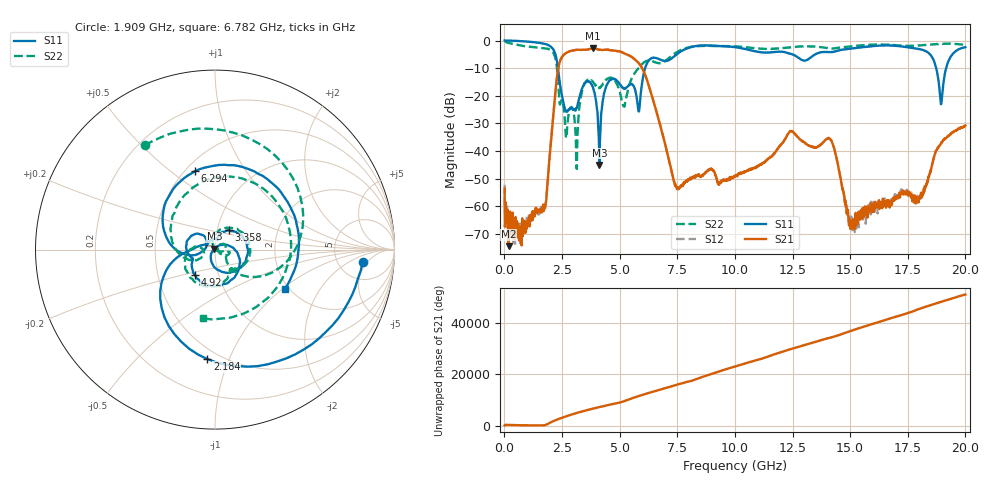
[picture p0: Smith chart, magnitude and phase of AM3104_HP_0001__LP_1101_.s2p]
!Created with skrf (http://scikit-rf.org).
# Hz S RI R 50.0
!freq ReS11 ImS11 ReS21 ImS21 ReS12 ImS12 ReS22 ImS22
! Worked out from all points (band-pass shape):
!   1601 points, 10 MHz to 20 GHz, reference 50 ohm
!   highest |S21| = -2.89 dB at 3.833 GHz (marker M1); lowest = -74.5 dB at 184.9 MHz (marker M2)
!   |S21| within 3 dB of the highest: 2.507 GHz to 5.513 GHz (3.006 GHz wide, 75 % of centre)
!   lowest |S11| = -45.0 dB at 4.12 GHz (marker M3), VSWR 1.01, Z = 49.7 + j0.448 ohm
!   |S11| at or under -10 dB: 2.323 GHz to 6.106 GHz (3.783 GHz wide, 89.8 % of centre); 18.74 GHz to 19.17 GHz (429.1 MHz wide, 2.26 % of centre)
!   |S22| runs from -46.5 to -0.2 dB; largest |S21 - S12| = 0.0069
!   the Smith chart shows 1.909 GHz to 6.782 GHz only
!   S11 on the Smith chart (normalised r, x): 1.909 GHz: 8.88, -3.80; 2.184 GHz: 0.43, -0.83; 3.358 GHz: 1.14, +0.25; 4.92 GHz: 0.77, -0.22; 6.294 GHz: 0.56, +0.61; 6.782 GHz: 1.90, -1.04
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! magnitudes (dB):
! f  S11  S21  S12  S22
! 10 MHz  0.0  -53.6  -52.2  -0.2
! 184.9 MHz  0.0  -74.5  -64.1  -0.9
! 1.909 GHz  -1.7  -47.5  -47.5  -3.1
! 2.184 GHz  -4.3  -21.1  -21.1  -5.6
! 2.684 GHz  -25.8  -4.5  -4.5  -35.3
! 3.346 GHz  -17.9  -3.4  -3.4  -19.2
! 3.358 GHz  -17.5  -3.4  -3.4  -18.6
! 3.833 GHz  -16.7  -2.9  -2.9  -14.9
! 4.12 GHz  -45.0  -3.4  -3.3  -17.1
! 4.92 GHz  -14.9  -3.9  -3.9  -16.6
! 5.82 GHz  -25.5  -8.1  -8.1  -10.0
! 6.294 GHz  -6.9  -17.1  -17.1  -7.3
! 6.682 GHz  -6.7  -28.3  -28.3  -8.2
! 6.782 GHz  -7.0  -31.4  -31.4  -8.2
! 7.506 GHz  -4.8  -53.3  -53.6  -4.0
! 10.01 GHz  -2.4  -49.2  -49.2  -2.1
! 13.34 GHz  -5.8  -38.6  -38.4  -2.2
! 14.19 GHz  -4.2  -36.3  -36.3  -2.9
! 15.04 GHz  -2.9  -65.8  -65.8  -2.1
! 16.68 GHz  -1.8  -57.9  -59.2  -1.6
! 18.95 GHz  -23.0  -37.2  -37.0  -1.2
! 20 GHz  -2.5  -30.8  -30.9  -1.5
